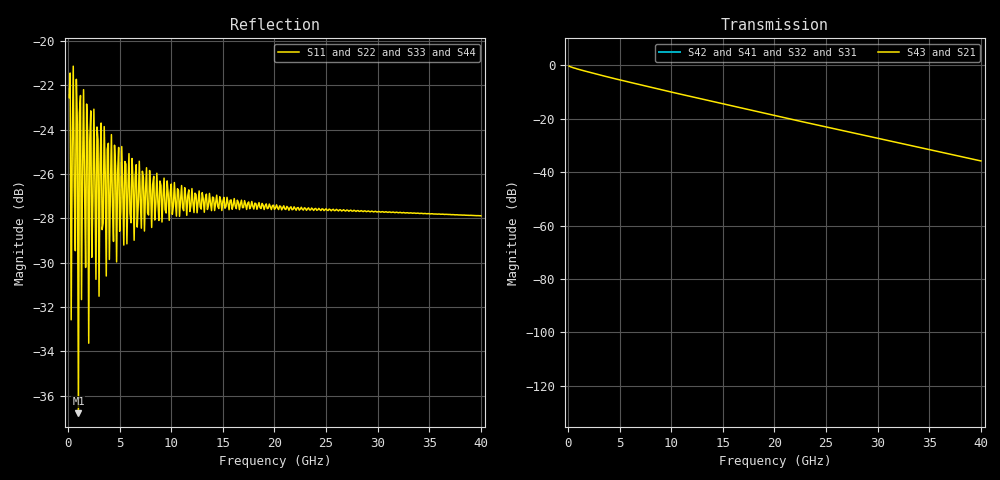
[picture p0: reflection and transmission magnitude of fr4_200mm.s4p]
! Touchstone Ver. 1.0
! Number of ports is 4
! port1 ->  port2
! port3 ->  port4
# Hz	S	RI	R	50.000000
! SCATTERING PARAMETERS  :
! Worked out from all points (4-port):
!   400 points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, 100 MHz to 40 GHz, reference 50 ohm
!   strongest paths, dB at 100 MHz, 10.1 GHz, 20.1 GHz, 30.1 GHz, 40 GHz:
!     S43: -0.3, -10.1, -18.9, -27.4, -35.8
!     S21: -0.3, -10.1, -18.9, -27.4, -35.8
!     S42: -, -, -, -, -
!     S41: -, -, -, -, -
!     S32: -, -, -, -, -
!     S31: -, -, -, -, -
!   lowest |S11| = -36.8 dB at 1 GHz (marker M1), VSWR 1.03, Z = 48.6 - j0.346 ohm
!   |S11| at or under -10 dB: start of sweep to end of sweep
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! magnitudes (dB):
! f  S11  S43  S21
! 100 MHz  -22.6  -0.3  -0.3
! 800 MHz  -21.7  -1.3  -1.3
! 1 GHz  -36.8  -1.5  -1.5
! 1.1 GHz  -23.3  -1.6  -1.6
! 1.5 GHz  -22.2  -2.0  -2.0
! 2 GHz  -33.6  -2.5  -2.5
! 40 GHz  -27.9  -35.8  -35.8
